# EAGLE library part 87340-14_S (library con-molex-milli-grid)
RECEPTACAL
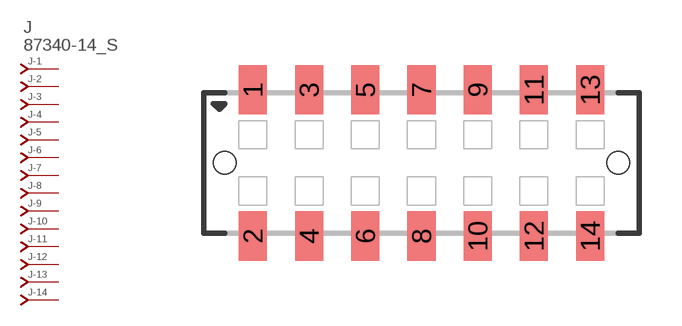
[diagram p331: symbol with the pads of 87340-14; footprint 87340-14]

Designator prefix J; gates -1=J-NV -2=J-N -3=J-N -4=J-N -5=J-N -6=J-N -7=J-N -8=J-N -9=J-N -10=J-N -11=J-N -12=J-N -13=J-N -14=J-N

## 87340-14_S  [87340-14]
1  -1:J  pas
2  -2:J  pas
3  -3:J  pas
4  -4:J  pas
5  -5:J  pas
6  -6:J  pas
7  -7:J  pas
8  -8:J  pas
9  -9:J  pas
10  -10:J  pas
11  -11:J  pas
12  -12:J  pas
13  -13:J  pas
14  -14:J  pas

## Footprint 87340-14 (pad centres in mm)
RECEPTACAL SMD Dual Row, Vertical, Low Profile
smd 1 x 1.75: 1 -6,2.6; 2 -6,-2.6; 3 -4,2.6; 4 -4,-2.6; 5 -2,2.6; 6 -2,-2.6; 7 0,2.6; 8 0,-2.6; 9 2,2.6; 10 2,-2.6; 11 4,2.6; 12 4,-2.6; 13 6,2.6; 14 6,-2.6
hole 0.8 at -7,0
hole 0.8 at 7,0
